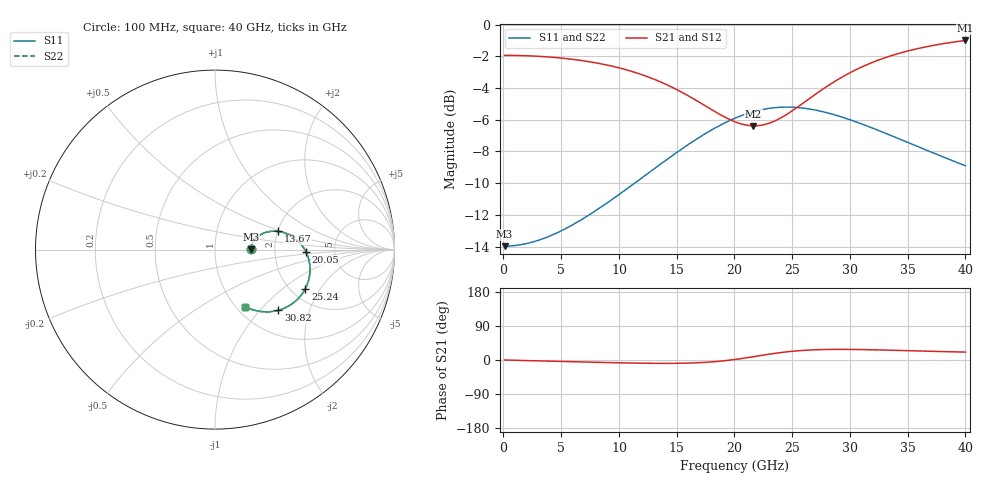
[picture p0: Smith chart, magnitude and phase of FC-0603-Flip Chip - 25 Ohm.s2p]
!Vishay Thin-Film
!FC Family
!Case Size 0603
!Assembly Style Flip Chip
!11/9/2015
!thinfilm@vishay.com
# GHz S MA R 50
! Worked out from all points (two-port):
!   101 points, 100 MHz to 40 GHz, reference 50 ohm
!   highest |S21| = -1.00 dB at 40 GHz (marker M1); lowest = -6.4 dB at 21.65 GHz (marker M2)
!   |S21| within 3 dB of the highest: start of sweep to 14.73 GHz; 27.81 GHz to end of sweep
!   lowest |S11| = -14.0 dB at 100 MHz (marker M3), VSWR 1.50, Z = 75 + j0.165 ohm
!   |S11| at or under -10 dB: start of sweep to 11.37 GHz
!   |S22| runs from -14.0 to -5.2 dB; largest |S21 - S12| = 0
!   S11 on the Smith chart (normalised r, x): 100 MHz: 1.50, +0.00; 13.67 GHz: 2.00, +0.47; 20.05 GHz: 3.05, -0.10; 25.24 GHz: 2.38, -1.48; 30.82 GHz: 1.43, -1.27; 40 GHz: 1.10, -0.80
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0.1  0.2 0.3  0.8 -0.1  0.8 -0.1  0.2 0.3
1.696  0.2028 5.1  0.7982 -1.3  0.7982 -1.3  0.2028 5.1
3.292  0.2103 9.4  0.7933 -2.5  0.7933 -2.5  0.2103 9.4
4.888  0.2225 13.1  0.7849 -3.7  0.7849 -3.7  0.2225 13.1
6.883  0.2441 16.5  0.7692 -5.2  0.7692 -5.2  0.2441 16.5
8.878  0.2723 18.4  0.7466 -6.6  0.7466 -6.6  0.2723 18.4
10.474  0.2994 18.7  0.7229 -7.6  0.7229 -7.6  0.2994 18.7
13.666  0.3644 16.2  0.6579 -8.9  0.6579 -8.9  0.3644 16.2
15.262  0.4009 13.3  0.6168 -8.6  0.6168 -8.6  0.4009 13.3
16.858  0.4384 9.4  0.5719 -7.2  0.5719 -7.2  0.4384 9.4
18.454  0.4747 4.4  0.528 -4.0  0.528 -4.0  0.4747 4.4
20.05  0.5067 -1.4  0.4936 1.4  0.4936 1.4  0.5067 -1.4
21.646  0.5312 -7.9  0.4793 8.7  0.4793 8.7  0.5312 -7.9
23.242  0.5457 -14.7  0.4921 16.4  0.4921 16.4  0.5457 -14.7
24.04  0.5488 -18.2  0.5083 19.7  0.5083 19.7  0.5488 -18.2
25.237  0.5483 -23.3  0.5419 23.6  0.5419 23.6  0.5483 -23.3
26.833  0.5391 -29.9  0.5963 26.8  0.5963 26.8  0.5391 -29.9
28.828  0.5173 -37.3  0.6666 28.0  0.6666 28.0  0.5173 -37.3
30.823  0.4889 -43.7  0.7293 27.6  0.7293 27.6  0.4889 -43.7
33.616  0.446 -51.0  0.7986 25.7  0.7986 25.7  0.446 -51.0
36.808  0.3994 -57.4  0.854 23.2  0.854 23.2  0.3994 -57.4
40  0.3587 -62.2  0.8913 20.9  0.8913 20.9  0.3587 -62.2
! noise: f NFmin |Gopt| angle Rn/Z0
0.1  6.472e-08  1  -1.941e-16  0.5
4.489  9.806e-08  1  -1.137e-14  0.5357
8.878  -1.929e-15  1  -1.909e-06  0.661
13.27  8.799e-08  1  8.356e-15  0.9614
17.66  -4.339e-15  1  -1.207e-06  1.622
22.05  1.918e-07  1  -8.239e-16  2.095
26.43  -9.643e-16  1  -8.538e-07  1.083
30.82  3.94e-08  1  -2.431e-14  0.4305
35.21  0  1  2.956e-15  0.1957
40  0  1  -1.207e-06  0.09684
